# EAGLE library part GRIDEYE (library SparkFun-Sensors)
Panasonic AMG8833 GRIDEye This 8x8 thermopile infrared sensor array allows for a low resolution thermal camera.
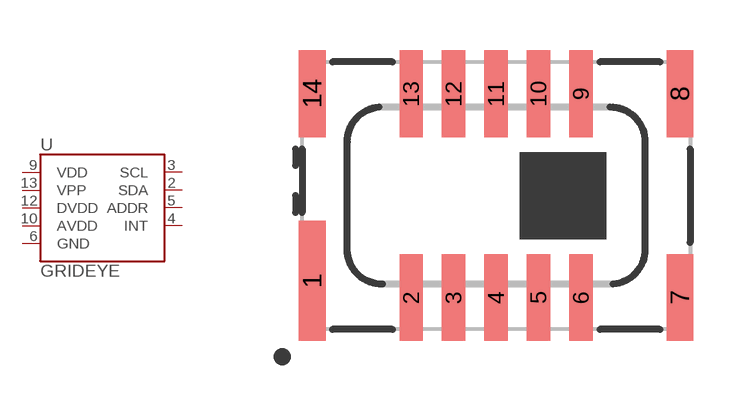
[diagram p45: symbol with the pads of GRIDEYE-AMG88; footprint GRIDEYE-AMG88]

Designator prefix U

## GRIDEYE (PROD_ID: IC-13912)  [GRIDEYE-AMG88]
2  SDA
3  SCL
4  INT
5  ADDR
6  GND
9  VDD
10  AVDD
12  DVDD
13  VPP

## Footprint GRIDEYE-AMG88 (pad centres in mm)
Panasonic AMG8833 GRIDEye Specifications: Pin count: 10 Pin pitch: .050 in. Area: .315 in. x 11.6 in. Datasheet referenced for footprint
smd 0.8 x 3.6: 1 -5.5,-2.55
smd 0.7 x 2.6: 2 -2.54,-3.05; 3 -1.27,-3.05; 4 0,-3.05; 5 1.27,-3.05; 6 2.54,-3.05; 9 2.54,3.05; 10 1.27,3.05; 11 0,3.05; 12 -1.27,3.05; 13 -2.54,3.05
smd 0.8 x 2.6: 7 5.5,-3.05; 8 5.5,3.05; 14 -5.5,3.05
